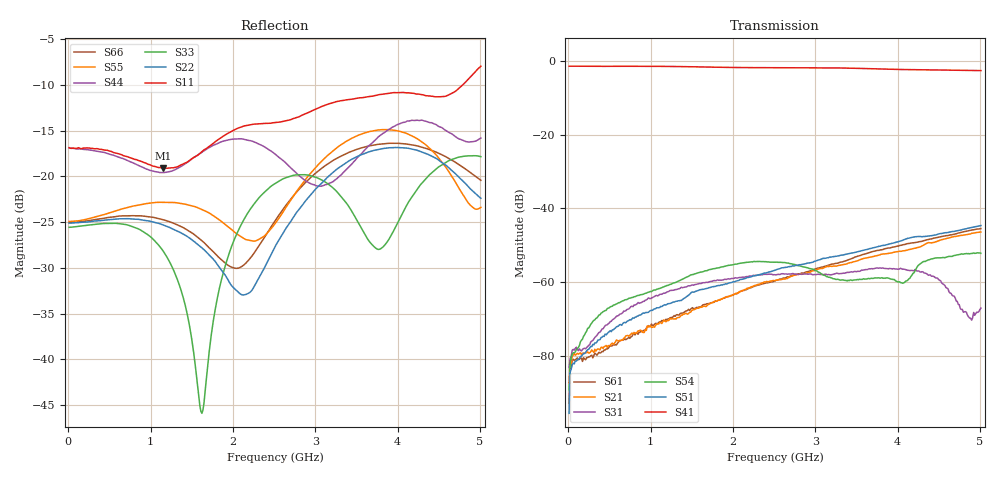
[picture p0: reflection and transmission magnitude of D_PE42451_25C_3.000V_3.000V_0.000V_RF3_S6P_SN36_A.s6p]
! Device ID: PE42451
! Serial: 36
! Insertion: A
! Temp: 25C
! VDD: 3.000
! Control_Hi: 100.000
! Control_Lo: 0.000
! Logic State: RF3
! Port 1: RFC
! Port 2: RF1
! Port 3: RF2
! Port 4: RF3
! Port 5: RF4
! Port 6: RF5
! V1 = 3.00
! V2 = 3.00
! V3 = 0.00
! V4 = 0.00
! IDD: 1.323780e-05
#  Hz  S  RI  R  50
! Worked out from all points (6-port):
!   401 points, 10 MHz to 5.01 GHz, reference 50 ohm
!   strongest paths, dB at 10 MHz, 1.26 GHz, 2.51 GHz, 3.76 GHz, 5.01 GHz:
!     S41: -1.5, -1.5, -1.9, -2.2, -2.7
!     S51: -95.5, -65.5, -56.8, -50.3, -44.6
!     S54: -89.1, -60.4, -54.5, -58.8, -52.1
!     S31: -83.1, -62.2, -58.0, -56.2, -67.0
!     S21: -87.2, -69.9, -59.6, -52.7, -46.4
!     S61: -92.8, -69.5, -59.6, -51.3, -45.5
!   lowest |S11| = -19.1 dB at 1.147 GHz (marker M1), VSWR 1.25, Z = 57.1 - j9.56 ohm
!   |S11| at or under -10 dB: start of sweep to 4.792 GHz
